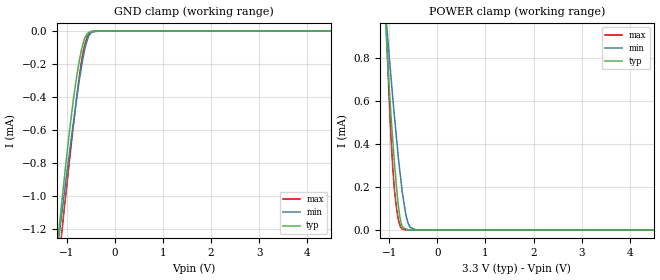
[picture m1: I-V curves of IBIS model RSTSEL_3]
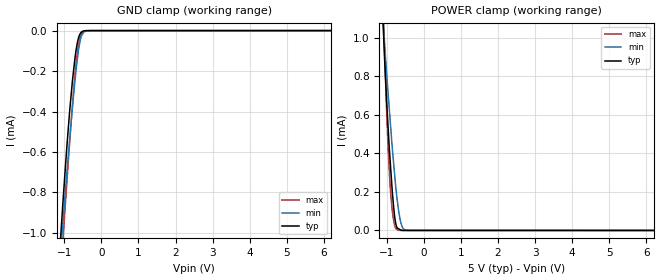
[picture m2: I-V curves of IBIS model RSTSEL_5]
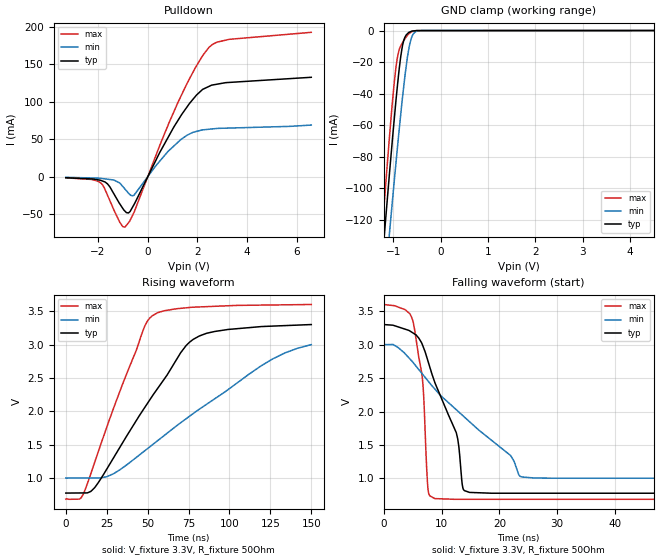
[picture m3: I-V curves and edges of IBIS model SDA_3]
|Texas Instruments Incorporated
|8-/10-/12-Bit, Octal-Channel, Ultra-Low Glitch, Voltage Output,
|   Two-Wire Interface DIGITAL-TO-ANALOG CONVERTERS
| Marketing part#   Voltage Range   Package-type   #pins
|DAC5578SPW   2.7V to 5.5V   TSSOP   16
|DAC5578SPWR   2.7V to 5.5V   TSSOP   16
|DAC5578SRGER   2.7V to 5.5V   VQFN   24
|DAC5578SRGET   2.7V to 5.5V   VQFN   24
|DAC6578SPW   2.7V to 5.5V   TSSOP   16
|DAC6578SPWR   2.7V to 5.5V   TSSOP   16
|DAC6578SRGER   2.7V to 5.5V   VQFN   24
|DAC6578SRGET   2.7V to 5.5V   VQFN   24
|DAC7578SPW   2.7V to 5.5V   TSSOP   16
|DAC7578SPWR   2.7V to 5.5V   TSSOP   16
|DAC7578SRGER   2.7V to 5.5V   VQFN   24
|DAC7578SRGET   2.7V to 5.5V   VQFN   24
[IBIS Ver]   4.0
[File name]   dacx578.ibs
[File Rev]   1.0
[Date]   06/08/2010
[Source]   Texas Instruments Incorporated.
   Analog-eLab, HPA
   12500 TI Blvd
   Dallas, TX -75243
   For Support e-mail: elab_ibis@list.ti.com
   Model geneated from simulations in TISPICE
[Notes]   Revision History:
   1.0: 07/26/2010
   - Initial version of the model
   - Initial Model generated from simulations in TISPICED
   - Specified temperature range = -40C to 125C. Maximum device power
   dissipation is 7.1 mW. Maximum theta ja (SO-8) = 118 C/W. IBIS
   test maximum temperature = 125C
   - Model names with a trailing _3 contains the model for
   3.3V (3.0V and 3.6V). Model names with trailing _5 contains
   the model for 5V (4.5V and 5.5V) operation.
   - Model not matched to measurements
   - C_comp although listed in numerical order of value are obtained
   from varying PVT conditions. For PVT conditions for each specific
   value refer the buffer description under respective [Model]. IBIS
   model user is responsible for using appropriate C_comp to simulate
   for Signal Integrity.
[Disclaimer]
 This model is designed as an aid for customers of Texas Instruments.
 No warranties, either expressed or implied, with respect to this third
 party software (if any) or with respect to its fitness for any
 particular purpose is claimed by Texas Instruments or the author. The
 software (if any) is provided solely on an "as is" basis. The entire
 risk as to its quality and performance is with the customer
[Copyright] (C) Copyright 2010 Texas Instruments Incorporated.
   All rights reserved.
|   DAC5578, DAC6578, and DAC7578 TTSOP package
[Component]   dacx578pw
[Manufacturer] TI
[Package]   |TTSOP-16 -  PW package
| variable   typ   min   max
R_pkg  0.055883   0.025700   0.075960
L_pkg  2.003210nH  1.377540nH  2.763480nH
C_pkg  0.279706pF  0.247630pF  0.339950pF
[Pin] signal_name  model_name  R_pin  L_pin C_pin
1   _LDAC   LDAC   0.06063  2.73325nH  0.33859pF
2   ADDR0   ADDRX   0.07090  2.04925nH  0.26777pF
3   AVDD   POWER   0.02570  1.37814nH  0.27361pF
4   VOUTA   TERM   0.04990  1.63284nH  0.24763pF
5   VOUTC   TERM   0.05564  1.74605nH  0.25294pF
6   VOUTE   TERM   0.05566  1.74724nH  0.25346pF
7   VOUTG   TERM   0.06562  1.94840nH  0.26228pF
8   VREFIN_VREFOUT   TERM   0.06170  2.76348nH  0.33995pF
9   _CLR   CLR   0.05843  2.69917nH  0.33694pF
10   VOUTH   TERM   0.06562  1.94850nH  0.26234pF
11   VOUTF   TERM   0.05566  1.74731nH  0.25347pF
12   VOUTD   TERM   0.05564  1.74612nH  0.25295pF
13   VOUTB   TERM   0.04990  1.63293nH  0.24763pF
14   GND   GND   0.02571  1.37754nH  0.27334pF
15   SDA   SDA   0.07596  2.15165nH  0.27271pF
16   SCLK   SCL   0.06145  2.74949nH  0.33968pF
|   DAC5578, DAC6578, and DAC7578 QFN package
[Component]   dacx578rge
[Manufacturer] TI
[Package]   |QFN-24  -  RGE package
| variable   typ   min   max
R_pkg  0.040021   0.000120   0.061170
L_pkg  0.694608nH  0.056080nH  1.040140nH
C_pkg  0.086353pF  0.037250pF  0.119350pF
[Pin] signal_name  model_name  R_pin  L_pin C_pin
1   NC   NC   0.00012  0.05927nH  0.03725pF
2   AVDD   POWER   0.02556  0.56969nH  0.11896pF
3   VOUTA   TERM   0.05112  0.85692nH  0.09616pF
4   VOUTC   TERM   0.05428  0.91391nH  0.09926pF
5   VOUTE   TERM   0.05128  0.86020nH  0.09557pF
6   VOUTG   TERM   0.05503  0.93123nH  0.09167pF
7   NC   NC   0.00012  0.05927nH  0.03725pF
8   VREFIN_VREFOUT   TERM   0.05294  0.88829nH  0.09712pF
9   RSTSEL   RSTSEL   0.04954  0.82551nH  0.09400pF
10   ADDR1   ADDRX   0.05128  0.85503nH  0.09649pF
11   ADDR0   ADDRX   0.05547  0.93077nH  0.10216pF
12   _CLR   CLR   0.06117  1.04014nH  0.09959pF
13   VOUTH   TERM   0.05503  0.92539nH  0.09187pF
14   VOUTF   TERM   0.05128  0.85339nH  0.09543pF
15   VOUTD   TERM   0.05429  0.90789nH  0.09911pF
16   VOUTB   TERM   0.05112  0.85007nH  0.09598pF
17   GND   GND   0.02556  0.56706nH  0.11935pF
18   NC   NC   0.00012  0.05927nH  0.03725pF
19   SDA   SDA   0.05896  0.99850nH  0.09669pF
20   SCLK   SCL   0.05374  0.89911nH  0.09941pF
21   TWOC   TWOC   0.05102  0.85017nH  0.09523pF
22   _LDAC   LDAC   0.05124  0.85416nH  0.09433pF
23   NC   NC   0.00012  0.05608nH  0.04508pF
24   NC   NC   0.00012  0.05927nH  0.03725pF
|   Model Selectors for RSTSEL, CLR, SDA, SCL, TWOC, LDAC,ADDRX
|Model names with a trailing _3 contains the model for
|   3.3V (3.0V and 3.6V).
|Model names with trailing _5 contains
|   the model for 5V (4.5V and 5.5V) operation.
[Model Selector]  RSTSEL
RSTSEL_3  3.3V digital input
RSTSEL_5  5V digital input
[Model Selector]  CLR
CLR_3  3.3V digital input
CLR_5  5V digital input
[Model Selector]  SDA
SDA_3  3.3V digital I/O_open_drain
SDA_5  5V digital I/O_open_drain
[Model Selector]  SCL
SCL_3  3.3V digital input
SCL_5  5V digital input
[Model Selector]  TWOC
TWOC_3  3.3V digital input
TWOC_5  5V digital input
[Model Selector]  LDAC
LDAC_3  3.3V digital input
LDAC_5  5V digital input
[Model Selector]  ADDRX
ADDRX_3  3.3V digital input
ADDRX_5  5V digital input
|   TERM Model
[Model] TERM
Model_type Terminator
C_comp   1e-20   1e-20   1e-20
| variable   typ   min   max
[Voltage Range]   3.3V   2.0V   5.5V
[POWER Clamp Reference]  3.3V   2.0V   5.5V
[GND Clamp Reference]   0.0V   0.0V   0.0V
|Operating Temperature
[Temperature Range]   27   85   -40
| Models and submodels in the file (15): TERM (Terminator), RSTSEL_3 (Input), RSTSEL_5 (Input), CLR_3 (Input), CLR_5 (Input), SDA_3 (I/O_open_drain), SDA_5 (I/O_open_drain), SCL_3 (Input), SCL_5 (Input), TWOC_3 (Input), TWOC_5 (Input), LDAC_3 (Input), LDAC_5 (Input), ADDRX_3 (Input), ADDRX_5 (Input)
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|   RSTSEL Model 3.3V MODEL
[Model] RSTSEL_3
Model_type   Input
Vinl = 0.99
Vinh = 2.31
|   typ   min   max
|   (Nom PVT)   (Fast PVT)  (Slow PVT)
C_comp   4.9429210e-13   4.7200600e-13   4.9507740e-13
|Where nom PVT is Nom process, 3.3V, 27C
|Fast PVT is Strong Process, 3.6V, -40C
|Slow PVT is Weak Process,   3.0V, 125C
[Voltage Range]   3.3   3   3.6
|Junction temperatures are used for [Temperature Range]
[Temperature Range]   27   125   -40
[Power Clamp Reference]   3.3   3   3.6
[GND Clamp Reference]   0   0   0
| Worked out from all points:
|   GND clamp passes 1 mA (typ) near -1.09 V on its own axis
|   POWER clamp passes 1 mA (typ) near -1.08 V on its own axis
[GND Clamp]
|   Voltage   I(typ)   I(min)   I(max)
-3.3V     -7.772mA   -6.534mA   -9.257mA
-1.173V   -1.23mA    -1.267mA   -1.412mA
-1.141V   -1.14mA    -1.19mA    -1.323mA
-1.12V    -1.08mA    -1.14mA    -1.264mA
-1.086V   -984.2uA   -1.062mA   -1.169mA
-932.5mV  -576.9uA   -707.4uA   -751.8uA
-801mV    -286.3uA   -421.5uA   -416.7uA
-665.6mV  -80.14uA   -167.8uA   -135.4uA
-605mV    -29.95uA   -84.25uA   -59.96uA
-541mV    -7.514uA   -28.19uA   -17.48uA
-345.6mV  -254.7nA   -205.3nA   -262.5nA
6.59V     0A         0A         0A
[POWER Clamp]
|   Voltage   I(typ)   I(min)   I(max)
-3.3V     13.6mA     10.98mA    16.4mA
-1.062V   904.8uA    974.4uA    939.1uA
-1.039V   807.3uA    907uA      810.7uA
-965.1mV  530.5uA    710.4uA    431.6uA
-922.7mV  399uA      600.1uA    270.4uA
-888.4mV  296.6uA    515.9uA    174.6uA
-838mV    168.6uA    396.8uA    80.73uA
-782.5mV  63.4uA     276.8uA    24.14uA
-734.7mV  19.53uA    183uA      4.619uA
-612.2mV  1.251uA    33.54uA    430.2nA
-443.6mV  265.7nA    419.5nA    420.2nA
6.59V     0A         0A         0A
|   RSTSEL Model 5V MODEL
[Model] RSTSEL_5
Model_type   Input
Vinl = 1.5
Vinh = 3.5
|   typ   min   max
|   (Nom PVT)   (Fast PVT)  (Slow PVT)
C_comp   4.7048420e-13   4.6177210e-13   4.7737260e-13
|Where nom PVT is Nom process, 5.0V, 27C
|Fast PVT is Strong Process, 5.5V, -40C
|Slow PVT is Weak Process,   4.5V, 125C
[Voltage Range]   5   4.5   5.5
[Temperature Range]   27   125   -40
|Junction temperatures are used for [Temperature Range]
[Power Clamp Reference]   5   4.5   5.5
[GND Clamp Reference]   0   0   0
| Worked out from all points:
|   GND clamp passes 1 mA (typ) near -1.09 V on its own axis
|   POWER clamp passes 1 mA (typ) near -1.08 V on its own axis
[GND Clamp]
|   Voltage   I(typ)   I(min)   I(max)
-5V       -13.1mA    -10.82mA   -15.79mA
-1.118V   -1.072mA   -1.136mA   -1.257mA
-1.053V   -892.6uA   -982.7uA   -1.074mA
-1.027V   -822.6uA   -924.1uA   -1.006mA
-853.8mV  -394.2uA   -533.9uA   -547.3uA
-782.2mV  -250.9uA   -382.4uA   -372.9uA
-711mV    -134.3uA   -246.2uA   -216.6uA
-671.7mV  -84.44uA   -176.4uA   -145uA
-608.1mV  -30.87uA   -86.63uA   -63.06uA
-549.6mV  -9.224uA   -33.4uA    -21.71uA
-493.8mV  -2.32uA    -12.19uA   -5.19uA
9.985V    0A         0A         0A
[POWER Clamp]
|   Voltage   I(typ)   I(min)   I(max)
-5V       23.59mA    19.04mA    28.46mA
-1.103V   1.088mA    1.091mA    1.184mA
-1.072V   942.8uA    1.003mA    994.2uA
-991.5mV  622.8uA    777.5uA    554.4uA
-956.8mV  506uA      689.8uA    396.4uA
-906.2mV  350.4uA    562.1uA    220.4uA
-866.3mV  239.7uA    461.5uA    127.7uA
-819.7mV  127.8uA    356.5uA    57.68uA
-735.9mV  20.35uA    185uA      4.811uA
-621.9mV  2.687uA    40.47uA    350.2nA
-434.5mV  236nA      320.5nA    344nA
9.985V    0A         0A         0A
|   SDA Model 3.3V MODEL
[Model] SDA_3
Model_type   I/O_open_drain
Polarity   Non-Inverting
Enable   Active-Low
Vinl = 0.99
Vinh = 2.31
Vmeas = 1.65
Vref = 1.65
Cref = 15pF
Rref = 50
|   typ   min   max
|   (Nom PVT)   (Fast PVT)  (Slow PVT)
C_comp   2.2456160e-12   1.8573770e-12   2.6552440e-12
|Where nom PVT is Nom process, 3.3V, 27C
|Fast PVT is Strong Process, 3.6V, -40C
|Slow PVT is Weak Process,   3.0V, 125C
[Voltage Range]   3.3   3   3.6
[Temperature Range]   27   125   -40
|Junction temperatures are used for [Temperature Range]
[Pullup Reference]   3.3   3   3.6
[Pulldown Reference]   0   0   0
[Power Clamp Reference]   3.3   3   3.6
[GND Clamp Reference]   0   0   0
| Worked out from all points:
|   slope of the pulldown table from 0 to 0.495 V, typ, clamps not added: 14.9 ohm
|   GND clamp passes 1 mA (typ) near -0.65 V on its own axis
|   falling waveform, V_fixture 3.3V, R_fixture 50Ohm: 20-80 % time 5.69ns typ, 14.8ns min, 1.66ns max; typ from 3.3 V to 0.778 V
|   rising waveform, V_fixture 3.3V, R_fixture 50Ohm: 20-80 % time 39.5ns typ, 66.8ns min, 26.4ns max; typ from 0.778 V to 3.3 V
[Pulldown]
|   Voltage   I(typ)   I(min)   I(max)
-3.3V     -1.428mA   -887uA     -1.602mA
-1.89V    -5.01mA    -2.295mA   -8.347mA
-1.531V   -13.34mA   -3.786mA   -31.57mA
-1.12V    -36.61mA   -8.654mA   -61.19mA
-920.1mV  -45.95mA   -16.41mA   -67.46mA
-774.5mV  -48.45mA   -22.05mA   -61.52mA
-559mV    -37.69mA   -24.88mA   -48.16mA
1.37V     83.14mA    50.46mA    109.7mA
1.967V    109mA      60.45mA    148.1mA
2.46V     120.4mA    63.3mA     172.4mA
3.271V    125.8mA    64.9mA     183.4mA
6.59V     132.7mA    68.92mA    192.8mA
[GND Clamp]
|   Voltage   I(typ)   I(min)   I(max)
-3.3V     -946.4mA   -916.5mA   -1.001A
-1.264V   -157.8mA   -190.9mA   -139.7mA
-1.223V   -142.8mA   -176.9mA   -123.2mA
-1.172V   -124.1mA   -159.6mA   -103.1mA
-1.077V   -89.85mA   -127.6mA   -66.59mA
-937.2mV  -42.98mA   -82.58mA   -22.3mA
-881.1mV  -26.49mA   -65.08mA   -12.92mA
-812.8mV  -11.1mA    -44.95mA   -8.17mA
-699.7mV  -2.055mA   -16.94mA   -3.066mA
-608.1mV  -385.6uA   -4.17mA    -716.8uA
-401.3mV  -34.15uA   -26.51uA   -53.65uA
6.59V     0A         0A         0A
[POWER Clamp]
|   SCR cell for ESD function. Effects occurr above VDD x 2
|   Voltage   I(typ)   I(min)   I(max)
-3.3V     0A         0A         0A
0V        0A         0A         0A
6.6V      0A         0A         0A
[Ramp]
R_load = 50
|   typ   min   max
dV/dt_r   1.51325/3.94388e-008   1.19869/6.66636e-008   1.74796/2.64223e-008
dV/dt_f   1.51325/5.68486e-009   1.19869/1.47579e-008   1.74796/1.66114e-009
[Falling Waveform]
V_fixture = 3.3V
V_fixture_min = 3V
V_fixture_max = 3.6V
R_fixture = 50Ohm
C_fixture = 0F
|   Time   V(typ)   V(min)   V(max)
0s        3.3V       3V         3.6V
5.044ns   3.175V     2.736V     3.353V
6.762ns   2.982V     2.552V     2.423V
7.683ns   2.745V     2.454V     817.8mV
8.852ns   2.43V      2.335V     697.9mV
12.54ns   1.684V     2.027V     686.8mV
13.67ns   862.4mV    1.939V     686.8mV
14.86ns   789.9mV    1.845V     686.8mV
26.04ns   778mV      1.006V     686.8mV
150ns     777.9mV    1.002V     686.7mV
[Rising Waveform]
V_fixture = 3.3V
V_fixture_min = 3V
V_fixture_max = 3.6V
R_fixture = 50Ohm
C_fixture = 0F
|   Time   V(typ)   V(min)   V(max)
0s        777.9mV    1.002V     686.7mV
10.6ns    779.8mV    1.004V     757.4mV
19.88ns   934.7mV    1.005V     1.399V
29.45ns   1.317V     1.071V     2.065V
47.58ns   2.034V     1.398V     3.237V
52.58ns   2.22V      1.494V     3.426V
73.46ns   2.984V     1.889V     3.55V
81.56ns   3.128V     2.033V     3.563V
126.5ns   3.277V     2.787V     3.593V
150ns     3.3V       3V         3.6V
